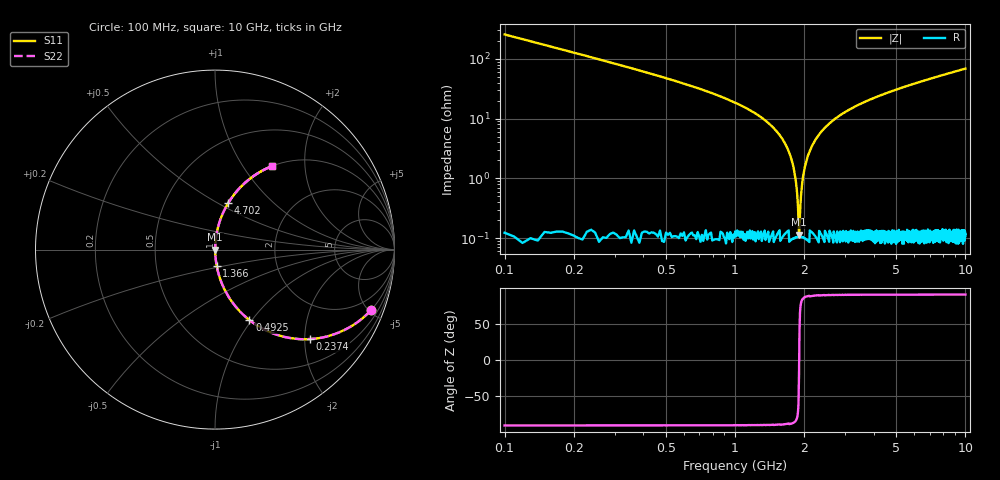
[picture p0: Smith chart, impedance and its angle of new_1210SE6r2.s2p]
!	AVX	Thin	Film	Operation	Date:	April 2007
!	Description:	Accu-P®	"Series,"	Thin	"Film,"	"SMD,"	RF	Capacitor
!	Part	Number:	12101J6R2BBT
!	100	MHz	-	5.05	GHz
!	Serial	Measurements
#	MHZ	S	MA	R	50
!	S11	S21	S12	S22
!	dB	Phase	dB	Phase	dB	Phase	dB	Phase
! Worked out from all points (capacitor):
!   1010 points, 100 MHz to 10 GHz, reference 50 ohm
!   read as one part in series: C = 6.2 pF near 149.1 MHz
!   lowest |Z| = 115 mohm at 1.896 GHz (marker M1)
!   series resonance near 1.899 GHz, so ESL is about 1.1 nH
!   S11 on the Smith chart (normalised r, x): 100 MHz: 1.01, -5.12; 237.4 MHz: 1.00, -2.13; 492.5 MHz: 1.00, -0.97; 1.366 GHz: 1.00, -0.18; 4.702 GHz: 1.00, +0.56; 10 GHz: 1.00, +1.37
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100  0.931 -21.3  0.364 68.6  0.364 68.6  0.931 -21.3
237.364  0.728 -43.2  0.684 46.8  0.684 46.8  0.728 -43.2
492.468  0.437 -64.0  0.899 25.9  0.899 25.9  0.437 -64.0
806.442  0.252 -75.2  0.967 14.6  0.967 14.6  0.252 -75.2
1365.709  0.09 -84.1  0.995 5.2  0.995 5.2  0.09 -84.1
1601.189  0.046 -86.0  0.998 2.6  0.998 2.6  0.046 -86.0
1758.176  0.021 -85.8  0.999 1.2  0.999 1.2  0.021 -85.8
1817.047  0.012 -84.0  0.999 0.7  0.999 0.7  0.012 -84.0
1866.105  0.00481 -76.5  0.999 0.3  0.999 0.3  0.00481 -76.5
1895.54  0.00119 -22.7  0.999 0.0  0.999 0.0  0.00119 -22.7
1934.787  0.00519 77.5  0.999 -0.3  0.999 -0.3  0.00519 77.5
1983.845  0.012 84.0  0.999 -0.7  0.999 -0.7  0.012 84.0
2042.716  0.02 85.7  0.999 -1.1  0.999 -1.1  0.02 85.7
2140.833  0.032 86.2  0.998 -1.9  0.998 -1.9  0.032 86.2
2268.385  0.048 85.9  0.998 -2.8  0.998 -2.8  0.048 85.9
2719.722  0.099 83.7  0.994 -5.7  0.994 -5.7  0.099 83.7
3406.541  0.165 80.1  0.985 -9.5  0.985 -9.5  0.165 80.1
4701.685  0.27 74.1  0.962 -15.6  0.962 -15.6  0.27 74.1
5054.906  0.295 72.6  0.954 -17.2  0.954 -17.2  0.295 72.6
6703.271  0.402 66.2  0.915 -23.7  0.915 -23.7  0.402 66.2
8351.635  0.491 60.5  0.87 -29.4  0.87 -29.4  0.491 60.5
10000  0.565 55.5  0.824 -34.4  0.824 -34.4  0.565 55.5
